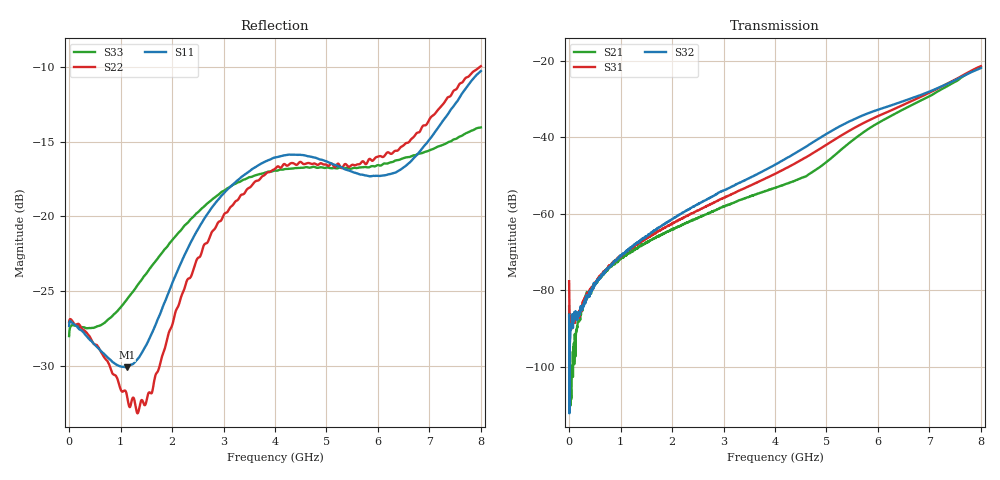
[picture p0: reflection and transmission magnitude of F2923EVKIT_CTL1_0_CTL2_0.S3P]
! Integrated Device Technology
! Corporate Headquarters
! 6024 Silver Creek Valley Road
! San Jose, CA 95138  USA
! Phone:  1-408-284-8200
! Toll Free:  1-800-223-1366
! Webpage:  http://www.idt.com/
! Timing and RF Division
! 515 Groton Road, Suite 102
! Westford, MA 01886-6024
! Device:  F2923
! Description: Constant Impedance Kz SP2T RF Switch
! Frequency:  0.3 MHz to 8 GHz
! Package:  4 mm x 4 mm QFN Plastic Package: 20 pin
! Ports:  3 RF, 3 DC
!  Pin  1  = GND
!  Pin  2  = GND
!  Pin  3  = RF1  = Port 1
!  Pin  4  = GND
!  Pin  5  = GND
!  Pin  6  = GND
!  Pin  7  = GND
!  Pin  8  = RF_COM  = Port 3
!  Pin  9  = GND
!  Pin  10  = GND
!  Pin  11  = GND
!  Pin  12  = GND
!  Pin  13  = RF2  = Port 2
!  Pin  14  = GND
!  Pin  15  = NC
!  Pin  16  = CTL2
!  Pin  17  = CTL1
!  Pin  18  = NC
!  Pin  19  = ModeCTL
!  Pin  20  = VCC
!  EP  = GND
! State:  All OFF
! Voltage:  VCC  = +3.3 V
!  CTL1  = 0 V (Logic LOW)
!  CTL2  = 0 V (Logic LOW)
! Data:  The device was measured on the F2923 EVKit
!  using a calibrated network analyzer.
!  The results below include the EVKit RF connector and
!		PCB loss effects. The reference plane is at
!  the SMA coaxial interface. Refer to the separate
!  measured thru line.s2p file for connector and PCB loss
!  and effects.
! Misc:
! Date Measured:  2017-8-14
! Date:  2017-8-14  SPJ
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# Hz S dB R 50
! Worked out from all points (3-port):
!   1601 points, 300 kHz to 8 GHz, reference 50 ohm
!   strongest paths, dB at 300 kHz, 2 GHz, 4 GHz, 6 GHz, 8 GHz:
!     S32: -86.3, -61.4, -47.1, -32.7, -21.8
!     S31: -77.6, -62.5, -49.5, -34.4, -21.3
!     S21: -84.2, -64.0, -53.2, -36.2, -21.5
!   lowest |S11| = -30.1 dB at 1.12 GHz (marker M1), VSWR 1.06, Z = 47.3 + j1.34 ohm
!   |S11| at or under -10 dB: start of sweep to end of sweep
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300000  -27.36 179.3  -80.45 -28.8  -83.00 -160.0
        -84.19 151.3  -27.09 178.7  -86.51 118.7
        -77.59 -149.5  -86.33 148.3  -28.02 179.5
3.952852e8  -28.24 160.2  -80.63 64.1  -80.69 54.6
            -80.60 60.9  -28.01 154.5  -80.72 51.2
            -80.53 53.1  -80.29 55.2  -27.48 172.1
1.120258e9  -30.11 153.1  -70.80 13.2  -69.84 17.3
            -70.58 11.9  -31.95 134.9  -69.54 25.2
            -69.87 17.9  -69.58 23.7  -25.58 161.5
1.60024e9  -27.89 157.8  -66.85 -23.0  -65.54 -12.3
           -66.78 -23.8  -31.85 151.3  -64.87 -5.7
           -65.56 -12.6  -64.81 -5.9  -23.35 147.2
2.755197e9  -19.50 115.6  -59.53 -111.0  -57.44 -94.6
            -59.51 -110.7  -21.18 113.0  -55.62 -91.6
            -57.42 -94.3  -55.64 -91.2  -18.95 97.6
4.00015e9  -16.07 46.1  -53.14 149.1  -49.52 169.7
           -53.15 148.9  -16.83 37.9  -47.13 168.0
           -49.50 169.7  -47.13 168.0  -16.95 34.6
5.480094e9  -17.00 -36.6  -41.03 39.0  -37.96 39.9
            -41.04 39.1  -16.60 -48.0  -35.53 23.4
            -37.96 39.9  -35.57 23.3  -16.82 -40.3
6.755047e9  -15.91 -100.6  -30.85 -106.8  -29.84 -94.5
            -30.85 -106.8  -14.43 -116.1  -29.27 -115.6
            -29.85 -94.5  -29.27 -115.6  -15.88 -115.2
7.415022e9  -12.87 -151.4  -26.02 176.5  -25.47 -165.7
            -26.03 176.5  -11.93 -163.0  -25.55 174.9
            -25.47 -165.8  -25.54 174.7  -14.99 -163.0
8e9  -10.28 149.9  -21.54 99.6  -21.36 123.6
     -21.55 99.6  -9.96 143.6  -21.85 106.5
     -21.34 123.5  -21.82 106.6  -14.06 146.2
